(* Oversampling SV ASDU data type (TwinCAT PLC little endian host byte order) *)
TYPE ST_SVASDU_IED_MUnn_LLN0_MSVCB02 : 
STRUCT
	nSmpCnt: ARRAY [0..cOversampleFactor_IED_MUnn_LLN0_MSVCB02_Asdu1-1] OF UINT; (* Sample counter *)
	eSmpSynch: ARRAY [0..cOversampleFactor_IED_MUnn_LLN0_MSVCB02_Asdu1-1] OF E_GseSvSmpSynch; (* Synchronization type: 0..2 *)
	tRefrTm: ARRAY [0..cOversampleFactor_IED_MUnn_LLN0_MSVCB02_Asdu1-1] OF T_UtcTime; (* Sample refresh time stamp (optional) *)
	
	IED_MUnn_InnATCTR1_AmpSv_instMag_i: ARRAY [0..cOversampleFactor_IED_MUnn_LLN0_MSVCB02_Asdu1-1] OF DINT;
	IED_MUnn_InnATCTR1_AmpSv_q: ARRAY [0..cOversampleFactor_IED_MUnn_LLN0_MSVCB02_Asdu1-1] OF ST_AcsiQuality;
	IED_MUnn_InnBTCTR2_AmpSv_instMag_i: ARRAY [0..cOversampleFactor_IED_MUnn_LLN0_MSVCB02_Asdu1-1] OF DINT;
	IED_MUnn_InnBTCTR2_AmpSv_q: ARRAY [0..cOversampleFactor_IED_MUnn_LLN0_MSVCB02_Asdu1-1] OF ST_AcsiQuality;
	IED_MUnn_InnCTCTR3_AmpSv_instMag_i: ARRAY [0..cOversampleFactor_IED_MUnn_LLN0_MSVCB02_Asdu1-1] OF DINT;
	IED_MUnn_InnCTCTR3_AmpSv_q: ARRAY [0..cOversampleFactor_IED_MUnn_LLN0_MSVCB02_Asdu1-1] OF ST_AcsiQuality;
	IED_MUnn_InnNTCTR4_AmpSv_instMag_i: ARRAY [0..cOversampleFactor_IED_MUnn_LLN0_MSVCB02_Asdu1-1] OF DINT;
	IED_MUnn_InnNTCTR4_AmpSv_q: ARRAY [0..cOversampleFactor_IED_MUnn_LLN0_MSVCB02_Asdu1-1] OF ST_AcsiQuality;
	IED_MUnn_UnnATVTR1_VolSv_instMag_i: ARRAY [0..cOversampleFactor_IED_MUnn_LLN0_MSVCB02_Asdu1-1] OF DINT;
	IED_MUnn_UnnATVTR1_VolSv_q: ARRAY [0..cOversampleFactor_IED_MUnn_LLN0_MSVCB02_Asdu1-1] OF ST_AcsiQuality;
	IED_MUnn_UnnBTVTR2_VolSv_instMag_i: ARRAY [0..cOversampleFactor_IED_MUnn_LLN0_MSVCB02_Asdu1-1] OF DINT;
	IED_MUnn_UnnBTVTR2_VolSv_q: ARRAY [0..cOversampleFactor_IED_MUnn_LLN0_MSVCB02_Asdu1-1] OF ST_AcsiQuality;
	IED_MUnn_UnnCTVTR3_VolSv_instMag_i: ARRAY [0..cOversampleFactor_IED_MUnn_LLN0_MSVCB02_Asdu1-1] OF DINT;
	IED_MUnn_UnnCTVTR3_VolSv_q: ARRAY [0..cOversampleFactor_IED_MUnn_LLN0_MSVCB02_Asdu1-1] OF ST_AcsiQuality;
	IED_MUnn_UnnNTVTR4_VolSv_instMag_i: ARRAY [0..cOversampleFactor_IED_MUnn_LLN0_MSVCB02_Asdu1-1] OF DINT;
	IED_MUnn_UnnNTVTR4_VolSv_q: ARRAY [0..cOversampleFactor_IED_MUnn_LLN0_MSVCB02_Asdu1-1] OF ST_AcsiQuality;
END_STRUCT
END_TYPE
